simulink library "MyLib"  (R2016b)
settings: Solver=VariableStepAuto  StartTime=0.0  StopTime=10.0  RelTol=1e-3
undefined symbols (not defined in the file or in its folder): dT, RngDwnLmt, RngUpLmt, T

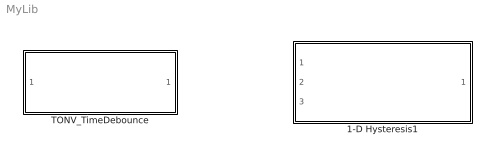
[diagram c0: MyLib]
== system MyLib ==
  1-D Hysteresis1 : Subsystem  TreatAsAtomicUnit=on  RTWFcnName=HysteresisCalc
  TONV_TimeDebounce : Subsystem  TreatAsAtomicUnit=on  RTWFcnName=TimeDebounce

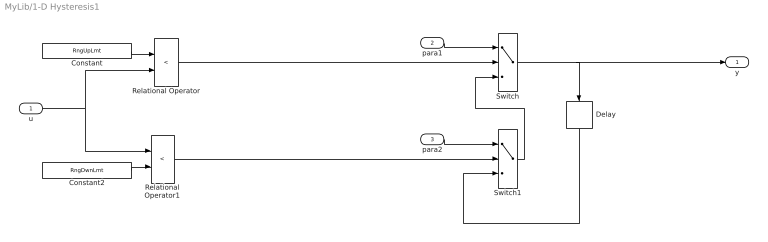
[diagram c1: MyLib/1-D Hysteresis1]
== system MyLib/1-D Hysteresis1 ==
  u : Inport
  para1 : Inport  Port=2
  para2 : Inport  Port=3
  Constant : Constant  Value=RngUpLmt
  Constant2 : Constant  Value=RngDwnLmt
  Delay : Delay  DelayLength=1  InitialCondition=0
  Relational Operator : RelationalOperator  Operator=<  OutDataTypeStr=boolean  RndMeth=Simplest
  Relational Operator1 : RelationalOperator  Operator=<  OutDataTypeStr=boolean  RndMeth=Simplest
  Switch : Switch  Criteria=u2 > Threshold
  Switch1 : Switch  Criteria=u2 > Threshold
  y : Outport
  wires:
  Relational Operator1/1 -> Switch1/2
  Relational Operator/1 -> Switch/2
  u/1 -> Relational Operator1/1, Relational Operator/2
  Switch/1 -> Delay/1, y/1
  Delay/1 -> Switch1/3
  Switch1/1 -> Switch/3
  para1/1 -> Switch/1
  para2/1 -> Switch1/1
  Constant/1 -> Relational Operator/1
  Constant2/1 -> Relational Operator1/2

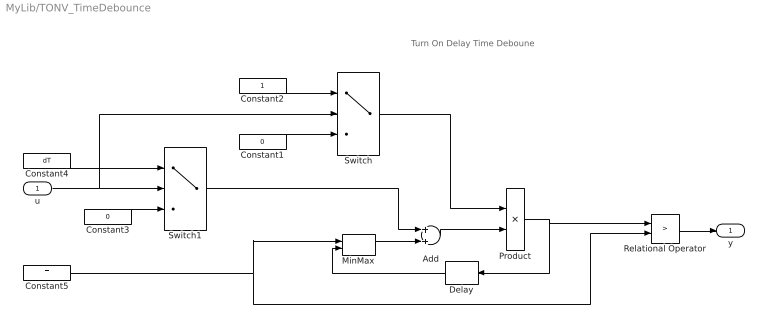
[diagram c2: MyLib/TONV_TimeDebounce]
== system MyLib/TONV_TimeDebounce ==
  note: Turn On Delay Time Deboune
  u : Inport
  Add : Sum
  Constant1 : Constant  Value=0  OutDataTypeStr=uint8
  Constant2 : Constant  OutDataTypeStr=uint8
  Constant3 : Constant  Value=0  OutDataTypeStr=single
  Constant4 : Constant  Value=dT  OutDataTypeStr=single
  Constant5 : Constant  Value=T  OutDataTypeStr=single
  Delay : Delay  DelayLength=1  InitialCondition=0
  MinMax : MinMax  Inputs=2
  Product : Product  OutMin=[0]  OutMax=[65535]  OutDataTypeStr=single
  Relational Operator : RelationalOperator  Operator=>  OutDataTypeStr=boolean  RndMeth=Simplest
  Switch : Switch  Criteria=u2 ~= 0
  Switch1 : Switch  Criteria=u2 ~= 0
  y : Outport
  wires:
  MinMax/1 -> Add/2
  Constant5/1 -> MinMax/1, Relational Operator/2
  Relational Operator/1 -> y/1
  Delay/1 -> MinMax/2
  Switch1/1 -> Add/1
  Product/1 -> Delay/1, Relational Operator/1
  Add/1 -> Product/2
  Constant1/1 -> Switch/3
  Constant2/1 -> Switch/1
  Constant3/1 -> Switch1/3
  Switch/1 -> Product/1
  u/1 -> Switch/2, Switch1/2
  Constant4/1 -> Switch1/1
